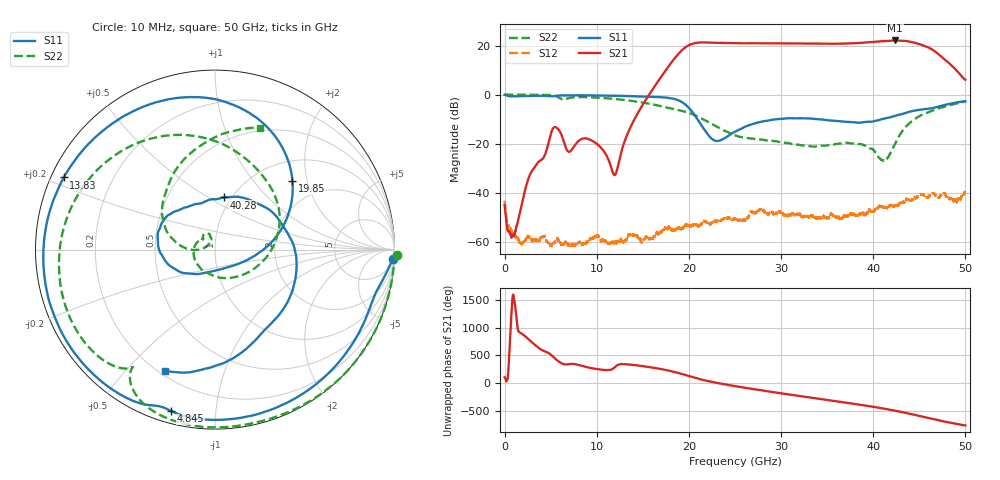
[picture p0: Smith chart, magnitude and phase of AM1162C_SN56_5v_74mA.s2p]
!Keysight Technologies,N5245B,MY58422270,A.16.20.02
!Date: Monday, June 03, 2024 23:21:32
!Correction: S11(C  2-Port  )
!S21(C  2-Port  )
!S12(C  2-Port  )
!S22(C  2-Port  )
!S2P File: Measurements: S11, S21, S12, S22:
# Hz S  dB  R 50
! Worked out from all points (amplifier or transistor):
!   6401 points, 10 MHz to 50 GHz, reference 50 ohm
!   highest |S21| = 22.1 dB at 42.36 GHz (marker M1)
!   |S21| within 3 dB of that: 19.55 GHz to 46.06 GHz (26.51 GHz wide, 80.8 % of centre)
!   unconditionally stable (mu >= 1): 267.6 MHz to 278.8 MHz; 289.2 MHz to 292.5 MHz; 2.143 GHz to end of sweep
!   at 8.336 GHz: K = 51.04, MAG = 1.3 dB, |S12| = -60.8 dB
!   at 25 GHz: K = 14.28, MAG = 21.2 dB, |S12| = -50.5 dB
!   at 50 GHz: K = 4.88, MAG = 12.8 dB, |S12| = -39.2 dB
!   S11 on the Smith chart (normalised r, x): 10 MHz: 6, -36; 4.845 GHz: 0.06, -0.76; 13.83 GHz: 0.04, +0.23; 19.85 GHz: 1.42, +1.63; 40.28 GHz: 0.92, +0.59; 50 GHz: 0.22, -0.65
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1e7  -0.08 -3.1  -44.99 103.7  -43.16 136.5  0.11 -1.6
4.84497e9  -0.61 -105.1  -18.57 175.8  -61.33 -109.8  -0.14 -100.8
8.34427e9  -0.25 -150.3  -18.08 -47.0  -60.94 -34.9  -0.98 -151.3
1.382755e10  -0.60 154.5  -11.97 -30.5  -56.71 162.4  -2.55 129.7
1.667854e10  -0.98 118.8  5.56 -98.5  -56.64 141.9  -4.42 89.0
1.844381e10  -1.75 83.9  14.72 -160.4  -55.20 -55.8  -5.92 62.6
1.984978e10  -4.78 41.6  19.81 133.1  -53.24 134.8  -7.24 36.9
2.096675e10  -10.19 6.3  21.16 79.3  -53.43 166.1  -8.95 13.0
2.242739e10  -17.77 -46.0  21.18 22.3  -52.30 118.4  -11.81 -20.0
2.5005e10  -15.06 -129.5  20.93 -56.8  -50.50 86.0  -16.53 -90.0
2.696555e10  -11.93 -155.7  20.90 -109.9  -48.12 -95.4  -17.91 -145.2
2.935569e10  -10.06 178.4  20.88 -171.0  -48.17 -124.5  -18.92 167.0
3.106629e10  -9.58 161.8  20.84 146.6  -49.17 29.9  -19.95 149.2
3.333927e10  -9.74 144.8  20.77 91.6  -49.58 26.0  -21.05 138.3
3.705728e10  -11.03 120.6  20.81 3.0  -49.43 -16.7  -19.52 124.6
4.027538e10  -10.61 80.5  21.53 -78.6  -46.14 -38.5  -23.68 108.2
4.167354e10  -9.35 52.9  21.92 -119.4  -45.35 107.3  -25.17 165.7
4.23609e10  -8.59 37.8  22.06 -141.5  -45.19 -167.8  -20.16 -179.2
4.373563e10  -7.14 2.8  21.76 170.6  -42.70 66.3  -12.32 166.1
4.536811e10  -5.98 -39.4  20.11 110.4  -40.60 20.9  -8.08 137.2
4.715682e10  -4.75 -72.2  16.25 41.2  -41.91 -20.7  -5.49 108.9
5e10  -2.72 -112.2  6.05 -49.3  -39.24 -61.9  -2.81 69.7
